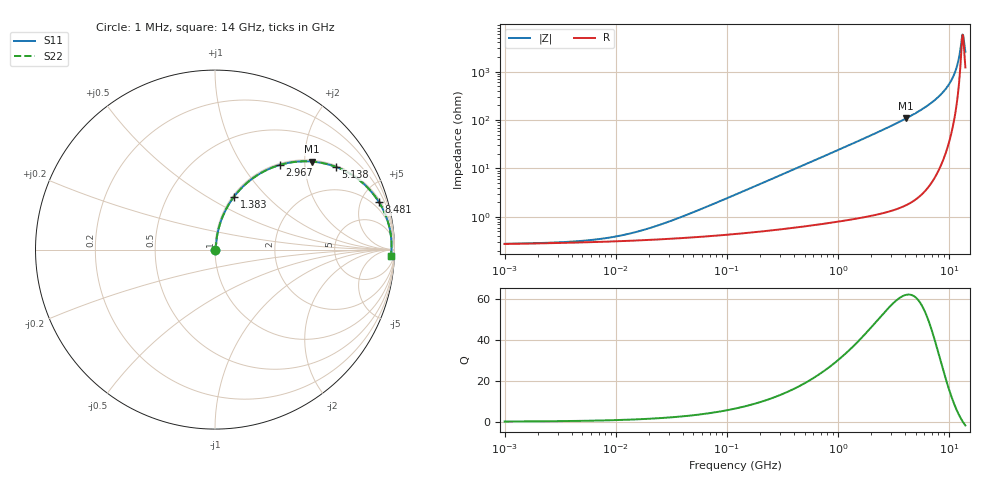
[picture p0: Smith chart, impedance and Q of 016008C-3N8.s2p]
# MHz S MA R 50
!Freq  MagS11  AngS11  MagS21  AngS21  MagS12  AngS12  MagS22  AngS22
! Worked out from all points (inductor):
!   801 points, 1 MHz to 14 GHz, reference 50 ohm
!   read as one part in series: L = 3.8 nH near 47.21 MHz
!   highest Q = 62.1 at 4.096 GHz (marker M1), where L = 4.2 nH
!   self-resonance near 13.19 GHz
!   S11 on the Smith chart (normalised r, x): 1 MHz: 1.01, +0.00; 1.383 GHz: 1.02, +0.67; 2.967 GHz: 1.03, +1.49; 5.138 GHz: 1.05, +2.89; 8.481 GHz: 1.24, +6.85; 14 GHz: 25, -45
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1  0.002771 4.9  0.9972 -0.0  0.9972 -0.0  0.002771 4.9
4.948533  0.00319 21.6  0.997 -0.1  0.997 -0.1  0.00319 21.6
11.14031  0.004118 39.9  0.9968 -0.2  0.9968 -0.2  0.004118 39.9
24.19749  0.006694 59.0  0.9966 -0.3  0.9966 -0.3  0.006694 59.0
119.742  0.0288 79.5  0.9952 -1.6  0.9952 -1.6  0.0288 79.5
289.5766  0.06885 81.5  0.9922 -3.9  0.9922 -3.9  0.06885 81.5
585.5183  0.138 79.3  0.9839 -7.9  0.9839 -7.9  0.138 79.3
1382.585  0.3141 70.2  0.9409 -18.3  0.9409 -18.3  0.3141 70.2
2025.523  0.4401 62.7  0.8886 -26.1  0.8886 -26.1  0.4401 62.7
2863.085  0.5779 53.7  0.8058 -35.3  0.8058 -35.3  0.5779 53.7
2967.442  0.593 52.6  0.7948 -36.4  0.7948 -36.4  0.593 52.6
4095.567  0.7283 42.3  0.6736 -46.7  0.6736 -46.7  0.7283 42.3
5137.888  0.8158 34.4  0.565 -54.7  0.565 -54.7  0.8158 34.4
6760.608  0.9019 24.4  0.4133 -64.4  0.4133 -64.4  0.9019 24.4
8481.181  0.9512 16.1  0.2774 -71.9  0.2774 -71.9  0.9512 16.1
9904.462  0.9723 10.5  0.1818 -76.0  0.1818 -76.0  0.9723 10.5
11027.44  0.9807 6.6  0.1153 -77.1  0.1153 -77.1  0.9807 6.6
11845.97  0.9835 4.0  0.07143 -74.6  0.07143 -74.6  0.9835 4.0
12725.26  0.9841 1.5  0.02991 -57.1  0.02991 -57.1  0.9841 1.5
13032.63  0.9837 0.6  0.01941 -32.8  0.01941 -32.8  0.9837 0.6
13507.66  0.9828 -0.7  0.02064 33.2  0.02064 33.2  0.9828 -0.7
14000  0.9813 -1.9  0.03822 59.7  0.03822 59.7  0.9813 -1.9
